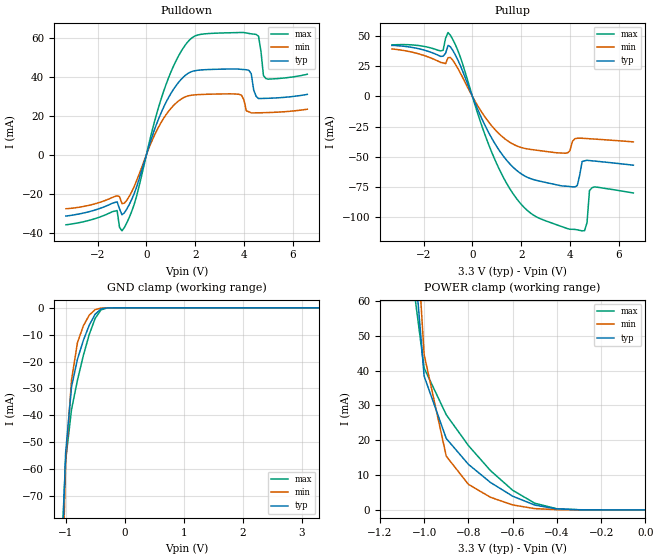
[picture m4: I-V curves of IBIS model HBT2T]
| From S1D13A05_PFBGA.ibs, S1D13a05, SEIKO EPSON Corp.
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[Model]   HBT2T
Model_type I/O
Enable Active-Low
Polarity Non-Inverting
Vinh=2.0
Vinl=0.8
C_comp   5p   4p   6p
[Temperature Range] 50   100   0
[Voltage Range]   3.3   3.0   3.6
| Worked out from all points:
|   slope of the pulldown table from 0 to 0.495 V, typ, clamps not added: 27.1 ohm
|   slope of the pullup table from 0 to 0.495 V, typ, clamps not added: 21.5 ohm
|   GND clamp passes 1 mA (typ) near -0.43 V on its own axis
|   POWER clamp passes 1 mA (typ) near -0.47 V on its own axis
[Pullup]
-3.3V     42.15mA    39.25mA    42.56mA
-1.3V     33.08mA    28.08mA    37.61mA
-900mV    41.01mA    32.19mA    50.49mA
1V        -41.53mA   -29.01mA   -55.83mA
2.5V      -68.74mA   -44.13mA   -98.09mA
3.9V      -74.3mA    -46.75mA   -109.3mA
4.2V      -74.89mA   -34.96mA   -110mA
4.6V      -53.23mA   -34.74mA   -111mA
4.7V      -52.84mA   -34.87mA   -104.3mA
4.8V      -53.04mA   -35mA      -77.92mA
4.9V      -53.23mA   -35.13mA   -75.58mA
6.6V      -56.86mA   -37.58mA   -79.82mA
[Pulldown]
-3.3V     -31.32mA   -27.59mA   -35.8mA
-1.2V     -24.05mA   -20.99mA   -28.51mA
-1.1V     -27.67mA   -21.42mA   -37.18mA
-900mV    -29.63mA   -24.72mA   -37.13mA
-400mV    -16.4mA    -13.21mA   -21.1mA
800mV     26.75mA    20.42mA    35.8mA
1.9V      42.8mA     30.61mA    60.2mA
3.8V      43.88mA    31mA       62.61mA
4.2V      43.29mA    22.07mA    62.14mA
4.5V      29.94mA    21.51mA    61.64mA
4.9V      28.92mA    21.61mA    39.05mA
6.6V      30.96mA    23.36mA    41.27mA
[GND Clamp]
-3.3V     -3.834A    -3.499A    -4.267A
-1.1V     -117.7mA   -143.2mA   -105.3mA
-1V       -53.96mA   -57.85mA   -56.85mA
-900mV    -29.39mA   -26.83mA   -37.84mA
-800mV    -19.14mA   -13mA      -26.98mA
-700mV    -12.14mA   -6.714mA   -17.76mA
-600mV    -6.473mA   -2.725mA   -9.921mA
-500mV    -2.364mA   -667uA     -3.937mA
-400mV    -431.6uA   -96.18uA   -746.3uA
-300mV    -40.31uA   -9.839uA   -57.18uA
3.3V      5.147nA    4.638uA    954.9pA
[POWER Clamp]
-3.3V     3.869A     3.537A     4.281A
-1.1V     115.6mA    148.9mA    90mA
-1V       38.44mA    44.67mA    40.76mA
-900mV    20.5mA     15.43mA    27.33mA
-800mV    13.09mA    7.333mA    18.49mA
-700mV    7.862mA    3.61mA     11.27mA
-600mV    3.928mA    1.413mA    5.634mA
-500mV    1.368mA    349.4uA    1.9mA
-400mV    257.4uA    50.44uA    302.4uA
-300mV    26.21uA    4.638uA    23.79uA
0V        5.147nA    5.009nA    1.16nA
[Ramp]
R_load=50
dV/dt_r   1.327E+0/2.525E-10   1.029E+0/3.370E-10   1.595E+0/2.072E-10
dV/dt_f   1.145E+0/3.943E-10   8.802E-1/5.208E-10   1.437E+0/2.936E-10
